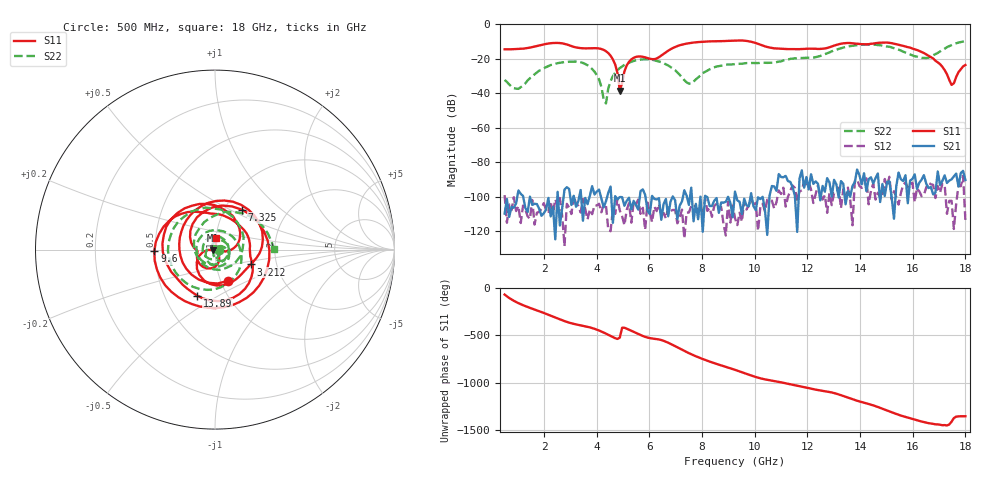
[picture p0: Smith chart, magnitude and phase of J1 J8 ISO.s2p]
!Agilent Technologies,N5230A,MY45001360,A.07.50.67
!Agilent N5230A: A.07.50.67
!Date: Tuesday, April 16, 2024 16:38:44
!Correction: S11(Full 2 Port(1,2))
!S21(Full 2 Port(1,2))
!S12(Full 2 Port(1,2))
!S22(Full 2 Port(1,2))
!S2P File: Measurements: S11, S21, S12, S22:
# Hz S  dB  R 50
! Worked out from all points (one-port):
!   201 points, 500 MHz to 18 GHz, reference 50 ohm
!   lowest |S11| = -38.4 dB at 4.875 GHz (marker M1), VSWR 1.02, Z = 48.9 - j0.346 ohm
!   |S11| at or under -10 dB: start of sweep to 8.076 GHz; 9.841 GHz to end of sweep
!   S11 on the Smith chart (normalised r, x): 500 MHz: 1.09, -0.39; 3.212 GHz: 1.47, -0.25; 7.325 GHz: 1.20, +0.58; 9.6 GHz: 0.49, -0.01; 13.89 GHz: 0.72, -0.40; 18 GHz: 1.00, +0.13
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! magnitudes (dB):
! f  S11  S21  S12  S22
! 500 MHz  -14.4  -109.8  -99.0  -32.2
! 1.025 GHz  -14.2  -96.4  -105.4  -37.4
! 2.075 GHz  -11.3  -107.5  -107.5  -24.8
! 3.212 GHz  -13.4  -105.8  -104.0  -21.6
! 3.475 GHz  -13.8  -113.9  -101.3  -22.4
! 4 GHz  -13.8  -97.1  -105.1  -29.4
! 4.35 GHz  -15.6  -102.6  -105.0  -45.9
! 4.438 GHz  -16.6  -97.7  -119.1  -37.1
! 4.7 GHz  -23.3  -99.7  -110.0  -28.0
! 4.875 GHz  -38.4  -100.2  -108.0  -25.3
! 5.05 GHz  -27.3  -105.2  -116.5  -23.5
! 5.312 GHz  -20.3  -107.3  -115.0  -21.7
! 6.362 GHz  -19.0  -100.9  -104.2  -21.5
! 7.325 GHz  -11.4  -96.3  -124.1  -32.3
! 9.25 GHz  -9.3  -97.0  -112.5  -23.0
! 9.6 GHz  -9.4  -101.1  -102.8  -22.6
! 12.22 GHz  -14.1  -92.5  -103.6  -19.3
! 13.89 GHz  -11.2  -84.2  -89.9  -12.0
! 15.11 GHz  -10.7  -91.0  -88.4  -12.9
! 16.77 GHz  -19.8  -98.6  -93.1  -18.0
! 17.48 GHz  -35.1  -89.9  -102.4  -11.9
! 18 GHz  -23.5  -90.3  -113.6  -9.7
